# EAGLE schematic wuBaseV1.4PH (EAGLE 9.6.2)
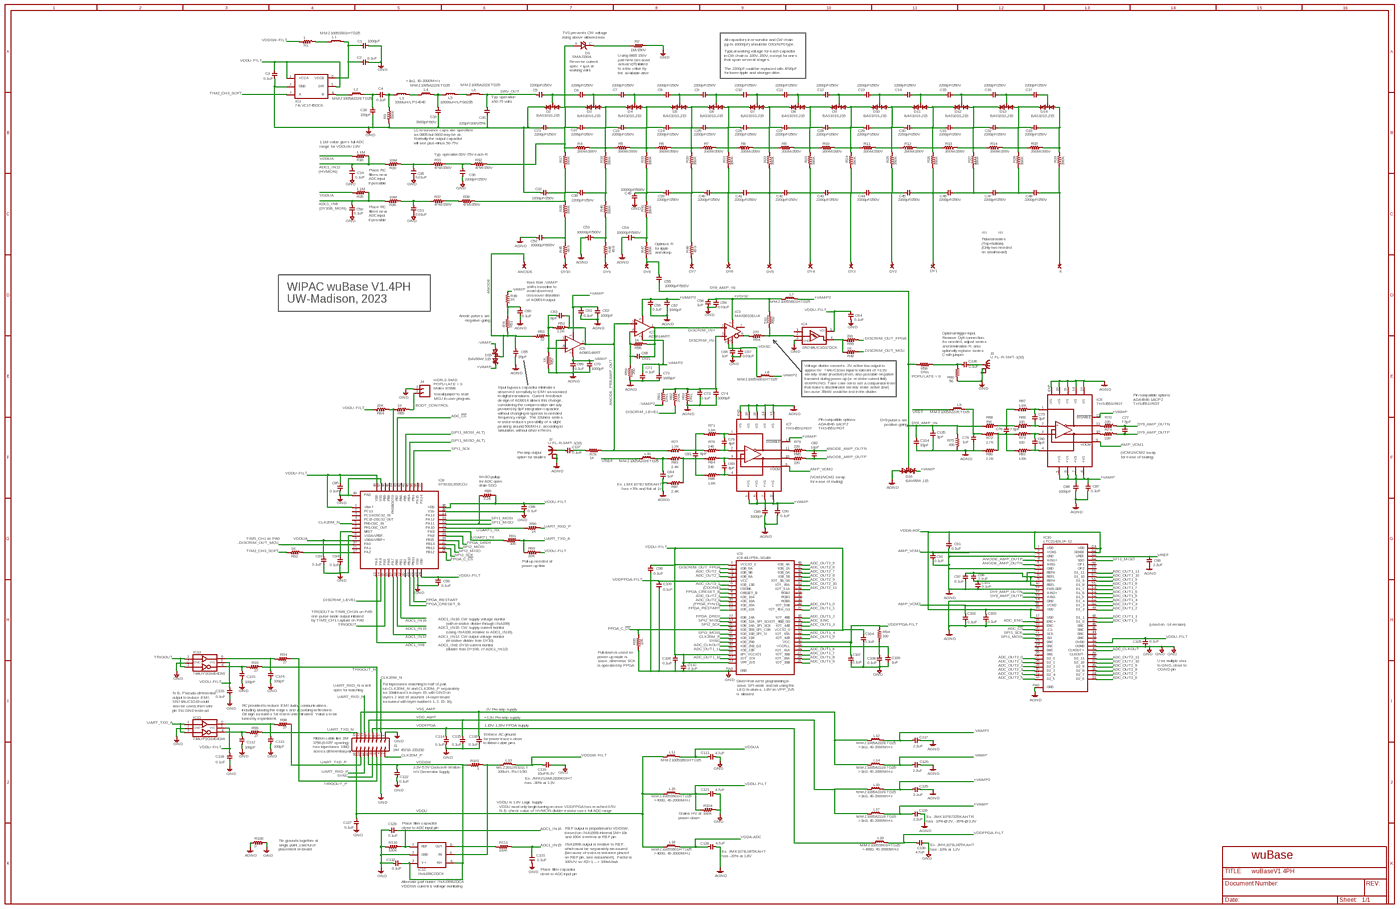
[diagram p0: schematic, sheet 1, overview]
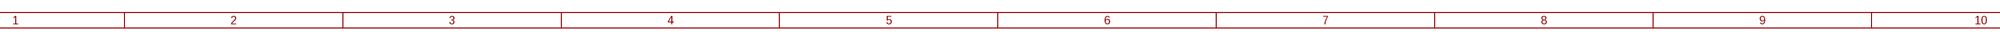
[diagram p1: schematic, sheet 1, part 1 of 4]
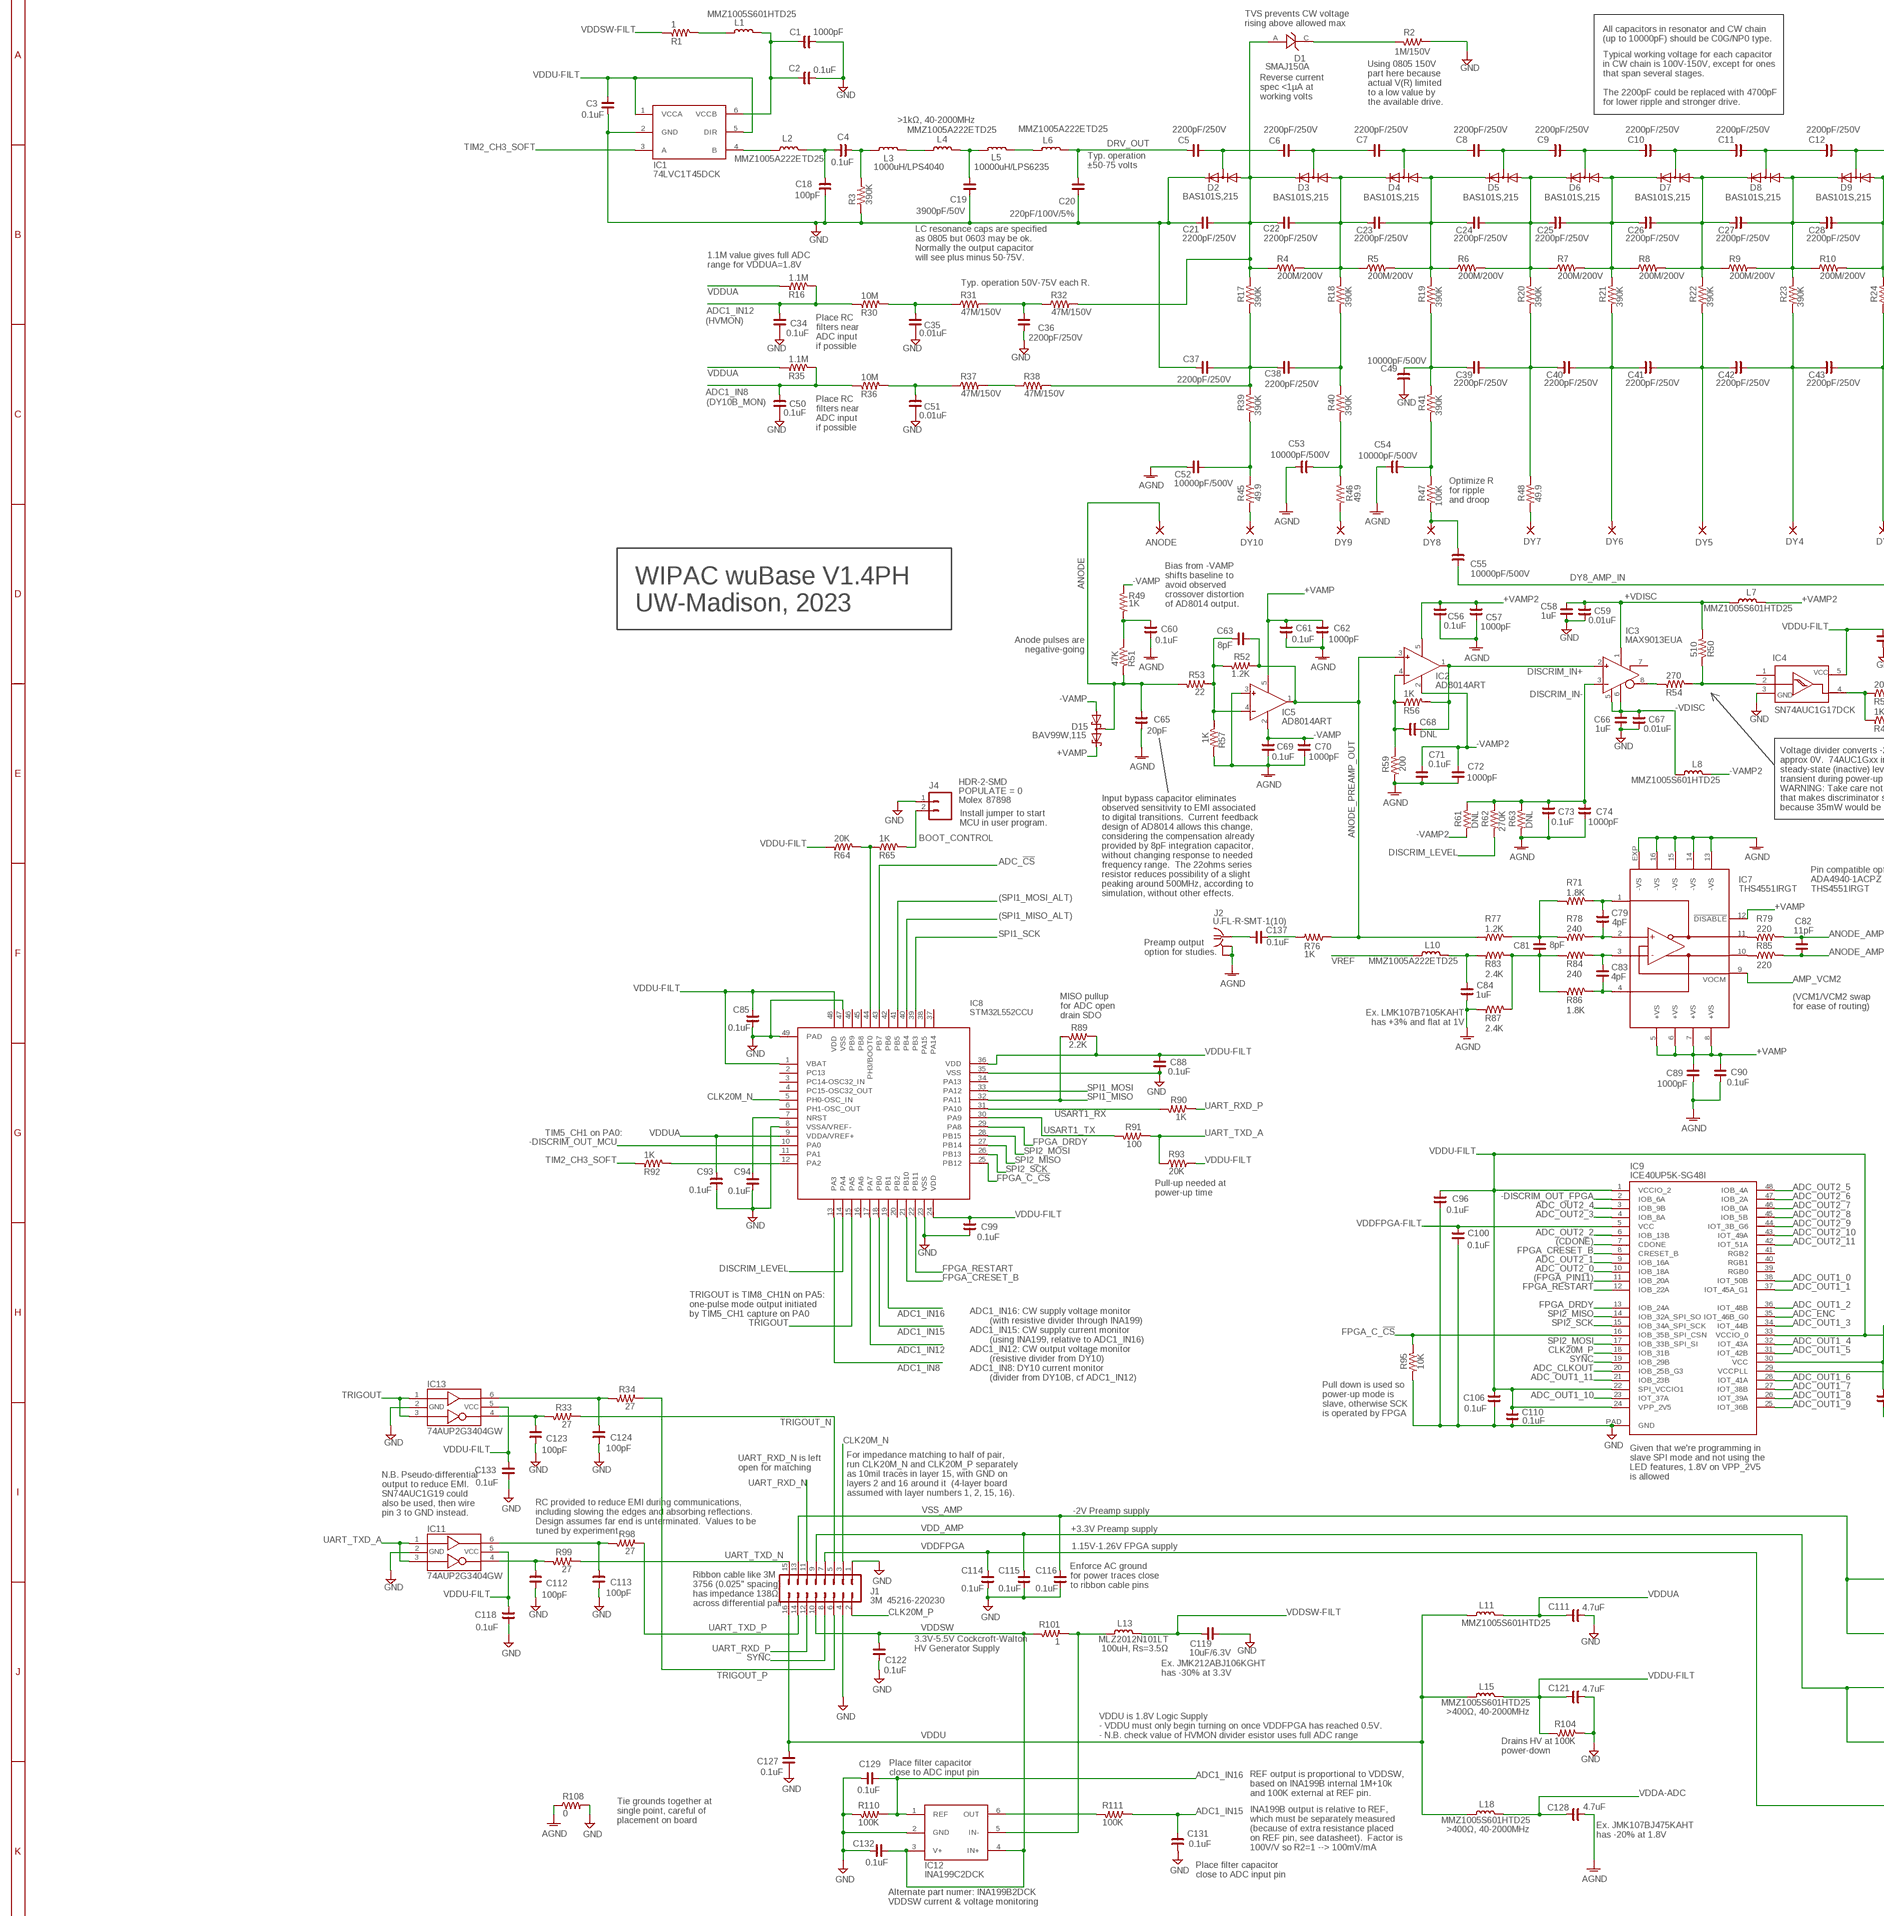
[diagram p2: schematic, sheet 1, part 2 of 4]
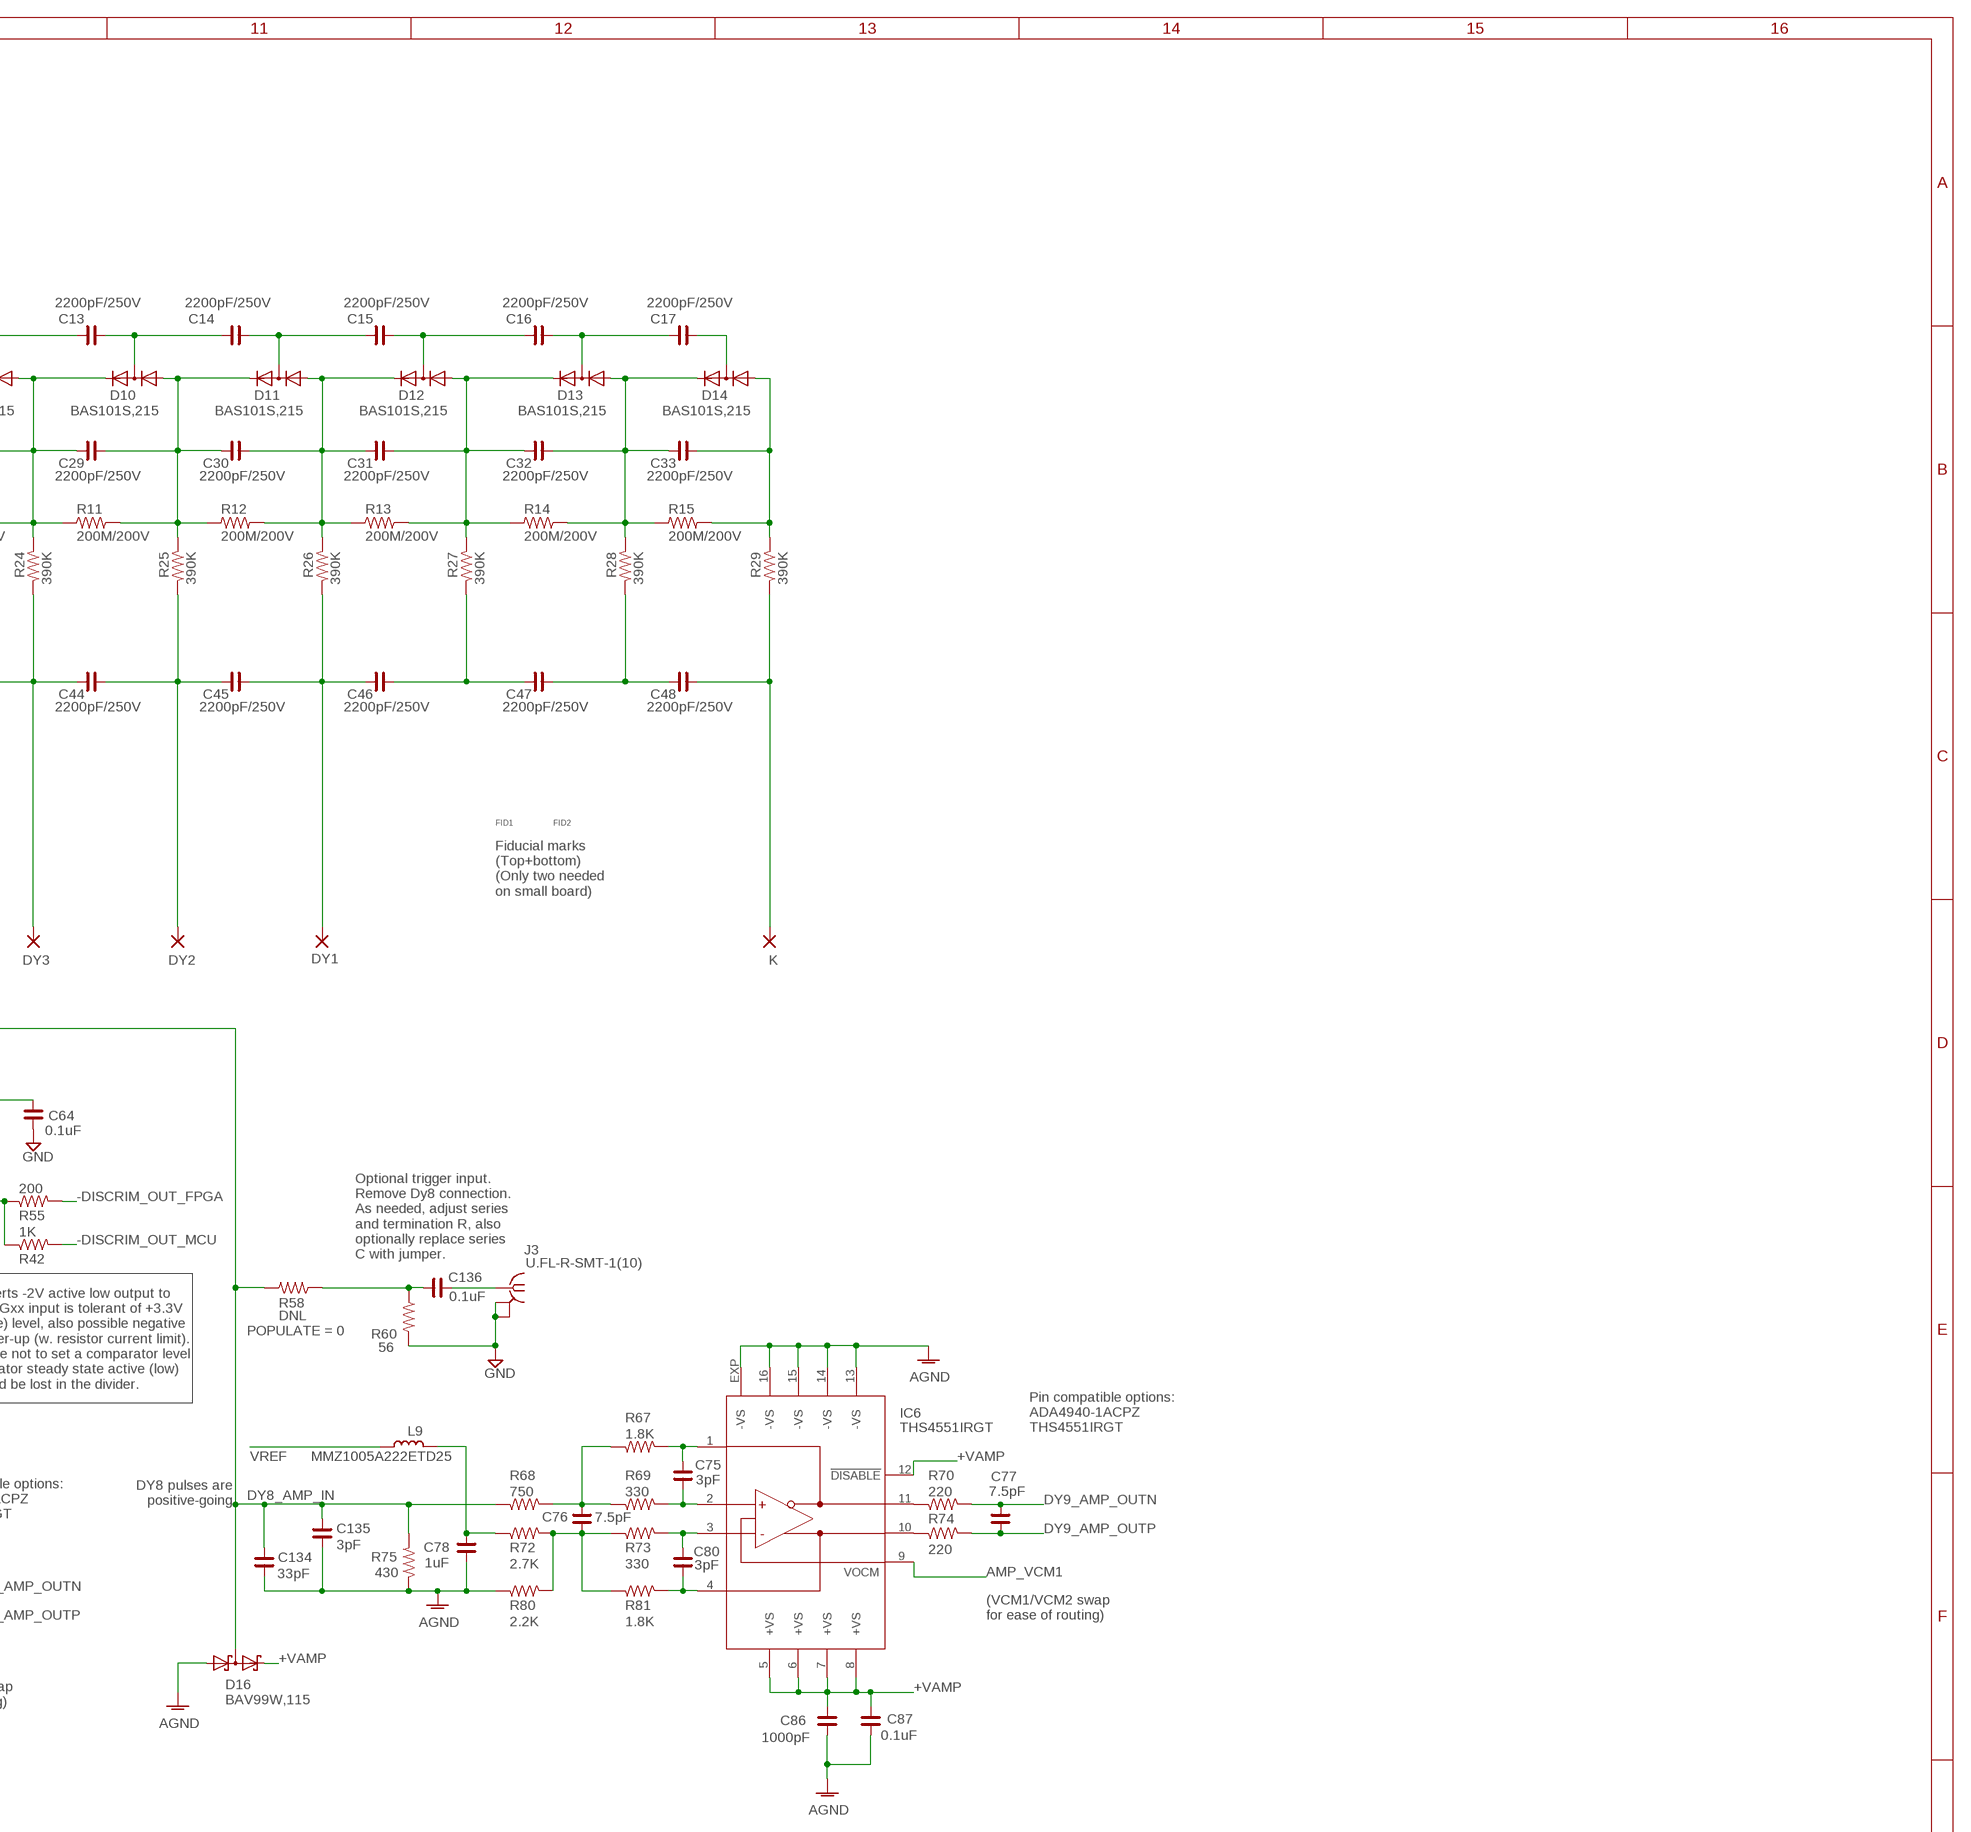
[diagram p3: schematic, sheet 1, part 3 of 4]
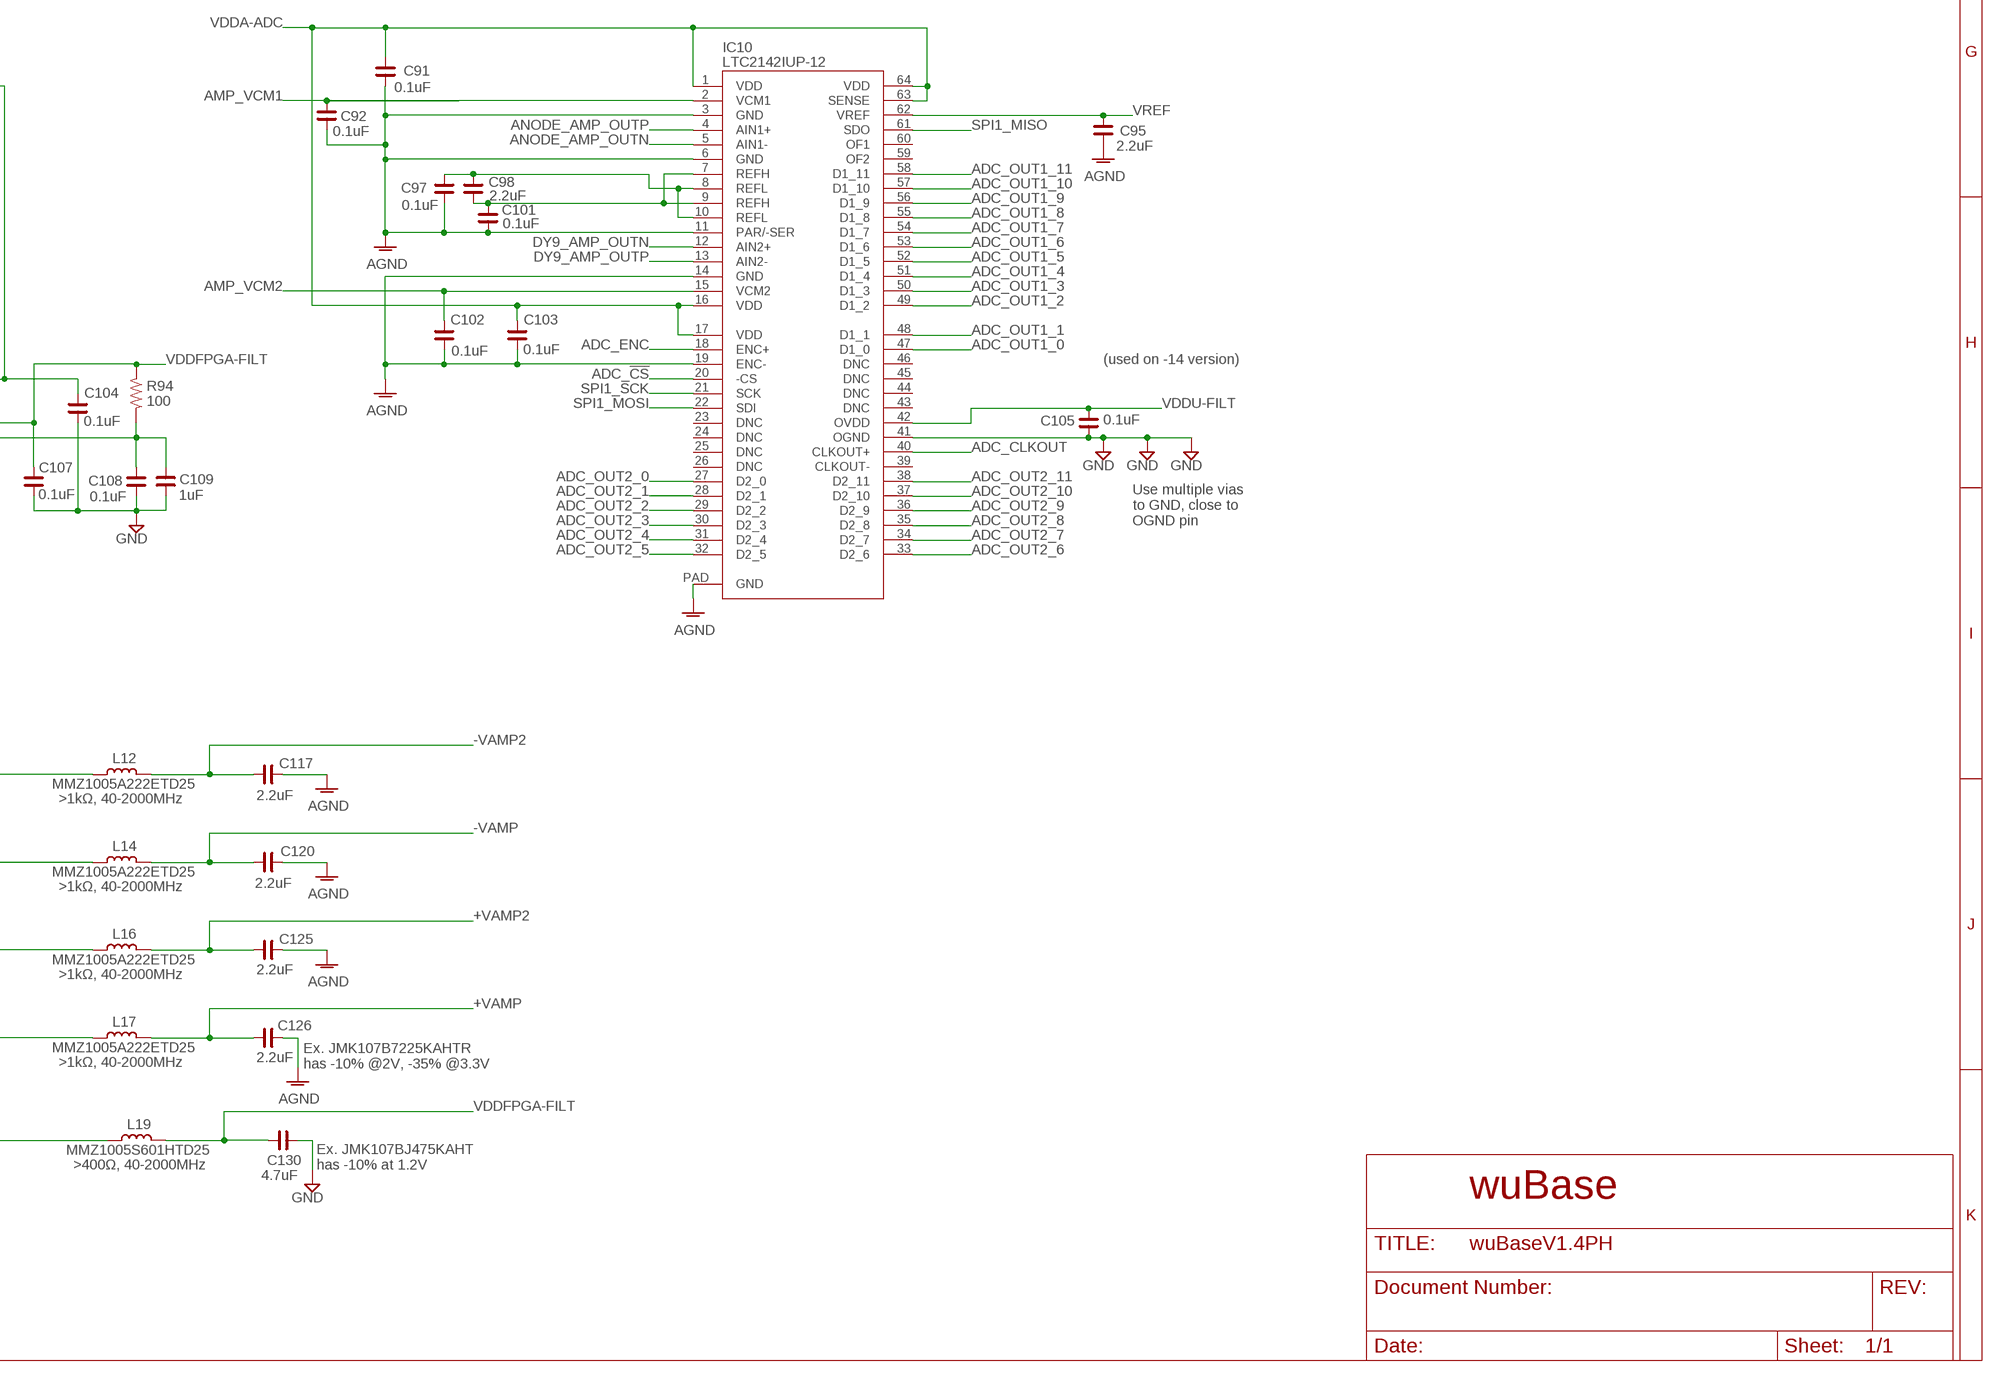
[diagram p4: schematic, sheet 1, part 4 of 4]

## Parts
ANODE  PAD-0430-BARE  [0430-BARE]
C1  1000pF  C_0402  [C0402]
C2  0.1uF  C_0402  [C0402]
C3  0.1uF  C_0402  [C0402]
C4  0.1uF  C_0402HV  [C0402-HV]
C5  2200pF/250V  C_0805HV  [C0805-HV]
C6  2200pF/250V  C_0805HV  [C0805-HV]
C7  2200pF/250V  C_0805HV  [C0805-HV]
C8  2200pF/250V  C_0805HV  [C0805-HV]
C9  2200pF/250V  C_0805HV  [C0805-HV]
C10  2200pF/250V  C_0805HV  [C0805-HV]
C11  2200pF/250V  C_0805HV  [C0805-HV]
C12  2200pF/250V  C_0805HV  [C0805-HV]
C13  2200pF/250V  C_0805HV  [C0805-HV]
C14  2200pF/250V  C_0805HV  [C0805-HV]
C15  2200pF/250V  C_0805HV  [C0805-HV]
C16  2200pF/250V  C_0805HV  [C0805-HV]
C17  2200pF/250V  C_0805HV  [C0805-HV]
C18  100pF  C_0402HV  [C0402-HV]
C19  3900pF/50V  C_0805HV  [C0805-HV]
C20  220pF/100V/5%  C_0805HV  [C0805-HV]
C21  2200pF/250V  C_0805HV  [C0805-HV]
C22  2200pF/250V  C_0805HV  [C0805-HV]
C23  2200pF/250V  C_0805HV  [C0805-HV]
C24  2200pF/250V  C_0805HV  [C0805-HV]
C25  2200pF/250V  C_0805HV  [C0805-HV]
C26  2200pF/250V  C_0805HV  [C0805-HV]
C27  2200pF/250V  C_0805HV  [C0805-HV]
C28  2200pF/250V  C_0805HV  [C0805-HV]
C29  2200pF/250V  C_0805HV  [C0805-HV]
C30  2200pF/250V  C_0805HV  [C0805-HV]
C31  2200pF/250V  C_0805HV  [C0805-HV]
C32  2200pF/250V  C_0805HV  [C0805-HV]
C33  2200pF/250V  C_0805HV  [C0805-HV]
C34  0.1uF  C_0402  [C0402]
C35  0.01uF  C_0402  [C0402]
C36  2200pF/250V  C_0805HV  [C0805-HV]
C37  2200pF/250V  C_0805HV  [C0805-HV]
C38  2200pF/250V  C_0805HV  [C0805-HV]
C39  2200pF/250V  C_0805HV  [C0805-HV]
C40  2200pF/250V  C_0805HV  [C0805-HV]
C41  2200pF/250V  C_0805HV  [C0805-HV]
C42  2200pF/250V  C_0805HV  [C0805-HV]
C43  2200pF/250V  C_0805HV  [C0805-HV]
C44  2200pF/250V  C_0805HV  [C0805-HV]
C45  2200pF/250V  C_0805HV  [C0805-HV]
C46  2200pF/250V  C_0805HV  [C0805-HV]
C47  2200pF/250V  C_0805HV  [C0805-HV]
C48  2200pF/250V  C_0805HV  [C0805-HV]
C49  10000pF/500V  C_1206HV  [C1206-HV]
C50  0.1uF  C_0402  [C0402]
C51  0.01uF  C_0402  [C0402]
C52  10000pF/500V  C_1206HV  [C1206-HV]
C53  10000pF/500V  C_1206HV  [C1206-HV]
C54  10000pF/500V  C_1206HV  [C1206-HV]
C55  10000pF/500V  C_1206HV  [C1206-HV]
C56  0.1uF  C_0402  [C0402]
C57  1000pF  C_0402  [C0402]
C58  1uF  C_0603  [C0603]
C59  0.01uF  C_0402  [C0402]
C60  0.1uF  C_0402  [C0402]
C61  0.1uF  C_0402  [C0402]
C62  1000pF  C_0402  [C0402]
C63  8pF  C_0402  [C0402]
C64  0.1uF  C_0402  [C0402]
C65  20pF  C_0402  [C0402]
C66  1uF  C_0603  [C0603]
C67  0.01uF  C_0402  [C0402]
C68  DNL  C_0402  [C0402]
C69  0.1uF  C_0402  [C0402]
C70  1000pF  C_0402  [C0402]
C71  0.1uF  C_0402  [C0402]
C72  1000pF  C_0402  [C0402]
C73  0.1uF  C_0402  [C0402]
C74  1000pF  C_0402  [C0402]
C75  3pF  C_0402  [C0402]
C76  7.5pF  C_0402  [C0402]
C77  7.5pF  C_0402  [C0402]
C78  1uF  C_0603  [C0603]
C79  4pF  C_0402  [C0402]
C80  3pF  C_0402  [C0402]
C81  8pF  C_0402  [C0402]
C82  11pF  C_0402  [C0402]
C83  4pF  C_0402  [C0402]
C84  1uF  C_0603  [C0603]
C85  0.1uF  C_0402  [C0402]
C86  1000pF  C_0402  [C0402]
C87  0.1uF  C_0402  [C0402]
C88  0.1uF  C_0402  [C0402]
C89  1000pF  C_0402  [C0402]
C90  0.1uF  C_0402  [C0402]
C91  0.1uF  C_0402  [C0402]
C92  0.1uF  C_0402  [C0402]
C93  0.1uF  C_0402  [C0402]
C94  0.1uF  C_0402  [C0402]
C95  2.2uF  C_0603  [C0603]
C96  0.1uF  C_0402  [C0402]
C97  0.1uF  C_0402  [C0402]
C98  2.2uF  C_0603  [C0603]
C99  0.1uF  C_0402  [C0402]
C100  0.1uF  C_0402  [C0402]
C101  0.1uF  C_0402  [C0402]
C102  0.1uF  C_0402  [C0402]
C103  0.1uF  C_0402  [C0402]
C104  0.1uF  C_0402  [C0402]
C105  0.1uF  C_0402  [C0402]
C106  0.1uF  C_0402  [C0402]
C107  0.1uF  C_0402  [C0402]
C108  0.1uF  C_0402  [C0402]
C109  1uF  C_0603  [C0603]
C110  0.1uF  C_0402  [C0402]
C111  4.7uF  C_0603  [C0603]
C112  100pF  C_0402  [C0402]
C113  100pF  C_0402  [C0402]
C114  0.1uF  C_0402  [C0402]
C115  0.1uF  C_0402  [C0402]
C116  0.1uF  C_0402  [C0402]
C117  2.2uF  C_0603  [C0603]
C118  0.1uF  C_0402  [C0402]
C119  10uF/6.3V  C_0805  [C0805]
C120  2.2uF  C_0603  [C0603]
C121  4.7uF  C_0603  [C0603]
C122  0.1uF  C_0402  [C0402]
C123  100pF  C_0402  [C0402]
C124  100pF  C_0402  [C0402]
C125  2.2uF  C_0603  [C0603]
C126  2.2uF  C_0603  [C0603]
C127  0.1uF  C_0402  [C0402]
C128  4.7uF  C_0603  [C0603]
C129  0.1uF  C_0402  [C0402]
C130  4.7uF  C_0603  [C0603]
C131  0.1uF  C_0402  [C0402]
C132  0.1uF  C_0402  [C0402]
C133  0.1uF  C_0402  [C0402]
C134  33pF  C_0402  [C0402]
C135  3pF  C_0402  [C0402]
C136  0.1uF  C_0402  [C0402]
C137  0.1uF  C_0402  [C0402]
D1  SMAJ150A  SMAJXXXA-HV  [DO214AC-HV]
D2  BAS101S,215  MMBD3004S-ROUNDED  [SOT23-ROUNDED]
D3  BAS101S,215  MMBD3004S-ROUNDED  [SOT23-ROUNDED]
D4  BAS101S,215  MMBD3004S-ROUNDED  [SOT23-ROUNDED]
D5  BAS101S,215  MMBD3004S-ROUNDED  [SOT23-ROUNDED]
D6  BAS101S,215  MMBD3004S-ROUNDED  [SOT23-ROUNDED]
D7  BAS101S,215  MMBD3004S-ROUNDED  [SOT23-ROUNDED]
D8  BAS101S,215  MMBD3004S-ROUNDED  [SOT23-ROUNDED]
D9  BAS101S,215  MMBD3004S-ROUNDED  [SOT23-ROUNDED]
D10  BAS101S,215  MMBD3004S-ROUNDED  [SOT23-ROUNDED]
D11  BAS101S,215  MMBD3004S-ROUNDED  [SOT23-ROUNDED]
D12  BAS101S,215  MMBD3004S-ROUNDED  [SOT23-ROUNDED]
D13  BAS101S,215  MMBD3004S-ROUNDED  [SOT23-ROUNDED]
D14  BAS101S,215  MMBD3004S-ROUNDED  [SOT23-ROUNDED]
D15  BAV99W,115  BAV99W  [SC70-3L]
D16  BAV99W,115  BAV99W  [SC70-3L]
DY1  PAD-0430-BARE  [0430-BARE]
DY2  PAD-0430-BARE  [0430-BARE]
DY3  PAD-0430-BARE  [0430-BARE]
DY4  PAD-0430-BARE  [0430-BARE]
DY5  PAD-0430-BARE  [0430-BARE]
DY6  PAD-0430-BARE  [0430-BARE]
DY7  PAD-0430-BARE  [0430-BARE]
DY8  PAD-0430-BARE  [0430-BARE]
DY9  PAD-0430-BARE  [0430-BARE]
DY10  PAD-0430-BARE  [0430-BARE]
FID1  FIDUCIAL_0.5MM  [FIDUCIAL_0.5MM]
FID2  FIDUCIAL_0.5MM  [FIDUCIAL_0.5MM]
IC1  74LVC1T45DCK  [SC70-6L-TI]
IC2  AD8014ART  [SOT23-5]
IC3  MAX9013EUA  [MSOP8]
IC4  SN74AUC1G17DCK  [SC70-5L-TI]
IC5  AD8014ART  [SOT23-5]
IC6  THS4551IRGT  ADA4940-1ACPZ  [LFCSP16]
IC7  THS4551IRGT  ADA4940-1ACPZ  [LFCSP16]
IC8  STM32L552CCU  [UFQFPN48-STMICRO]
IC9  ICE40UP5K-SG48I  [QFN48-ICE40ULTRA]
IC10  LTC2142IUP-12  LTC2141-12UP  [QFN64-LTC214X]
IC11  74AUP2G3404GW  [SC70-6L-TI]
IC12  INA199C2DCK  INA199B2DCK  [SC70-6L-TI]
IC13  74AUP2G3404GW  [SC70-6L-TI]
J1  HDR-16  HDR-2X8-3M-45216-220230  [3M-45216-220230]
J2  COAX-2GNDU.FL  [HIROSE_U.FL-R-SMT-1]
J3  COAX-2GNDU.FL  [HIROSE_U.FL-R-SMT-1]
J4  HDR-2-SMD  [HEADER-SMD-2X1-MINIMUM]
K  PAD-0430-BARE  [0430-BARE]
L1  MMZ1005S601HTD25  L_0402  [L0402]
L2  MMZ1005A222ETD25  L_0402HV  [L0402-HV]
L3  1000uH/LPS4040  L_LPS4040-REDUCED  [LPS4040-REDUCED]
L4  MMZ1005A222ETD25  L_0402HV  [L0402-HV]
L5  10000uH/LPS6235  L_LPS6235-REDUCED  [LPS6235-REDUCED]
L6  MMZ1005A222ETD25  L_0402HV  [L0402-HV]
L7  MMZ1005S601HTD25  L_0402  [L0402]
L8  MMZ1005S601HTD25  L_0402  [L0402]
L9  MMZ1005A222ETD25  L_0402  [L0402]
L10  MMZ1005A222ETD25  L_0402  [L0402]
L11  MMZ1005S601HTD25  L_0402  [L0402]
L12  MMZ1005A222ETD25  L_0402  [L0402]
L13  MLZ2012N101LT  L_0805  [L0805]
L14  MMZ1005A222ETD25  L_0402  [L0402]
L15  MMZ1005S601HTD25  L_0402  [L0402]
L16  MMZ1005A222ETD25  L_0402  [L0402]
L17  MMZ1005A222ETD25  L_0402  [L0402]
L18  MMZ1005S601HTD25  L_0402  [L0402]
L19  MMZ1005S601HTD25  L_0402  [L0402]
R1  1  R_0402  [R0402]
R2  1M/150V  R_0805HV  [R0805-HV]
R3  390K  R_0402HV  [R0402-HV]
R4  200M/200V  R_1206HV  [R1206-HV]
R5  200M/200V  R_1206HV  [R1206-HV]
R6  200M/200V  R_1206HV  [R1206-HV]
R7  200M/200V  R_1206HV  [R1206-HV]
R8  200M/200V  R_1206HV  [R1206-HV]
R9  200M/200V  R_1206HV  [R1206-HV]
R10  200M/200V  R_1206HV  [R1206-HV]
R11  200M/200V  R_1206HV  [R1206-HV]
R12  200M/200V  R_1206HV  [R1206-HV]
R13  200M/200V  R_1206HV  [R1206-HV]
R14  200M/200V  R_1206HV  [R1206-HV]
R15  200M/200V  R_1206HV  [R1206-HV]
R16  1.1M  R_0402  [R0402]
R17  390K  R_0402HV  [R0402-HV]
R18  390K  R_0402HV  [R0402-HV]
R19  390K  R_0402HV  [R0402-HV]
R20  390K  R_0402HV  [R0402-HV]
R21  390K  R_0402HV  [R0402-HV]
R22  390K  R_0402HV  [R0402-HV]
R23  390K  R_0402HV  [R0402-HV]
R24  390K  R_0402HV  [R0402-HV]
R25  390K  R_0402HV  [R0402-HV]
R26  390K  R_0402HV  [R0402-HV]
R27  390K  R_0402HV  [R0402-HV]
R28  390K  R_0402HV  [R0402-HV]
R29  390K  R_0402HV  [R0402-HV]
R30  10M  R_0402  [R0402]
R31  47M/150V  R_0805HV  [R0805-HV]
R32  47M/150V  R_0805HV  [R0805-HV]
R33  27  R_0402  [R0402]
R34  27  R_0402  [R0402]
R35  1.1M  R_0402  [R0402]
R36  10M  R_0402  [R0402]
R37  47M/150V  R_0805HV  [R0805-HV]
R38  47M/150V  R_0805HV  [R0805-HV]
R39  390K  R_0402HV  [R0402-HV]
R40  390K  R_0402HV  [R0402-HV]
R41  390K  R_0402HV  [R0402-HV]
R42  1K  R_0402  [R0402]
R45  49.9  R_0402HV  [R0402-HV]
R46  49.9  R_0402HV  [R0402-HV]
R47  100K  R_0402HV  [R0402-HV]
R48  49.9  R_0402HV  [R0402-HV]
R49  1K  R_0402  [R0402]
R50  510  R_0402  [R0402]
R51  47K  R_0402  [R0402]
R52  1.2K  R_0402  [R0402]
R53  22  R_0402  [R0402]
R54  270  R_0402  [R0402]
R55  200  R_0402  [R0402]
R56  1K  R_0402  [R0402]
R57  1K  R_0402  [R0402]
R58  DNL  R_0402  [R0402]
R59  200  R_0402  [R0402]
R60  56  R_0402  [R0402]
R61  DNL  R_0402  [R0402]
R62  270K  R_0402  [R0402]
R63  DNL  R_0402  [R0402]
R64  20K  R_0402  [R0402]
R65  1K  R_0402  [R0402]
R67  1.8K  R_0402  [R0402]
R68  750  R_0402  [R0402]
R69  330  R_0402  [R0402]
R70  220  R_0402  [R0402]
R71  1.8K  R_0402  [R0402]
R72  2.7K  R_0402  [R0402]
R73  330  R_0402  [R0402]
R74  220  R_0402  [R0402]
R75  430  R_0402  [R0402]
R76  1K  R_0402  [R0402]
R77  1.2K  R_0402  [R0402]
R78  240  R_0402  [R0402]
R79  220  R_0402  [R0402]
R80  2.2K  R_0402  [R0402]
R81  1.8K  R_0402  [R0402]
R83  2.4K  R_0402  [R0402]
R84  240  R_0402  [R0402]
R85  220  R_0402  [R0402]
R86  1.8K  R_0402  [R0402]
R87  2.4K  R_0402  [R0402]
R89  2.2K  R_0402  [R0402]
R90  1K  R_0402  [R0402]
R91  100  R_0402  [R0402]
R92  1K  R_0402  [R0402]
R93  20K  R_0402  [R0402]
R94  100  R_0402  [R0402]
R95  10K  R_0402  [R0402]
R98  27  R_0402  [R0402]
R99  27  R_0402  [R0402]
R101  1  R_0402  [R0402]
R104  100K  R_0402  [R0402]
R108  0  R_0402  [R0402]
R110  100K  R_0402  [R0402]
R111  100K  R_0402  [R0402]

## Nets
(CDONE): IC9.7(CDONE)
(FPGA_PIN11): IC9.11(IOB_20A)
(SPI1_MISO_ALT): IC8.40(PB4)
(SPI1_MOSI_ALT): IC8.41(PB5)
+VAMP: C61.1 C62.1 C86.1 C87.1 C89.1 C90.1 C126.2 D15.2(C2) D16.2(C2) IC5.5(V+) IC6.5(+VS) IC6.6(+VS) IC6.7(+VS) IC6.8(+VS) IC6.12(!DISABLE) IC7.5(+VS) IC7.6(+VS) IC7.7(+VS) IC7.8(+VS) IC7.12(!DISABLE) L17.2
+VAMP2: C56.1 C57.1 C125.2 IC2.5(V+) L7.2 L16.2
+VDISC: C58.1 C59.1 IC3.1(VCC) L7.1 R50.2
-DISCRIM_BUFOUT: IC4.4(OUT) R42.1 R55.1
-DISCRIM_OUT: IC3.8(QBAR) R54.1
-DISCRIM_OUT_DIVIDER: IC4.2(IN) R50.1 R54.2
-DISCRIM_OUT_FPGA: IC9.2(IOB_6A) R55.2
-DISCRIM_OUT_MCU: IC8.10(PA0) R42.2
-VAMP: C69.1 C70.1 C120.2 D15.1(A1) IC5.2(V-) L14.2 R49.1
-VAMP2: C71.1 C72.1 C117.2 IC2.2(V-) L8.2 L12.2 R61.2
-VDISC: C66.1 C67.1 IC3.5(LE) IC3.6(GND) L8.1
ADC1_IN8: C50.1 IC8.13(PA3) R35.2 R36.1
ADC1_IN12: C34.1 IC8.17(PA7) R16.2 R30.1
ADC1_IN15: C131.2 IC8.18(PB0) R111.1
ADC1_IN16: C129.2 IC8.19(PB1) IC12.1(REF) R110.1
ADC_!CS: IC8.43(PB7) IC10.20(-CS)
ADC_CLKOUT: IC9.20(IOB_25B_G3) IC10.40(CLKOUT+)
ADC_ENC: IC9.35(IOT_46B_G0) IC10.18(ENC+)
ADC_OUT1_0: IC9.38(IOT_50B) IC10.47(D1_0)
ADC_OUT1_1: IC9.37(IOT_45A_G1) IC10.48(D1_1)
ADC_OUT1_2: IC9.36(IOT_48B) IC10.49(D1_2)
ADC_OUT1_3: IC9.34(IOT_44B) IC10.50(D1_3)
ADC_OUT1_4: IC9.32(IOT_43A) IC10.51(D1_4)
ADC_OUT1_5: IC9.31(IOT_42B) IC10.52(D1_5)
ADC_OUT1_6: IC9.28(IOT_41A) IC10.53(D1_6)
ADC_OUT1_7: IC9.27(IOT_38B) IC10.54(D1_7)
ADC_OUT1_8: IC9.26(IOT_39A) IC10.55(D1_8)
ADC_OUT1_9: IC9.25(IOT_36B) IC10.56(D1_9)
ADC_OUT1_10: IC9.23(IOT_37A) IC10.57(D1_10)
ADC_OUT1_11: IC9.21(IOB_23B) IC10.58(D1_11)
ADC_OUT2_0: IC9.10(IOB_18A) IC10.27(D2_0)
ADC_OUT2_1: IC9.9(IOB_16A) IC10.28(D2_1)
ADC_OUT2_2: IC9.6(IOB_13B) IC10.29(D2_2)
ADC_OUT2_3: IC9.4(IOB_8A) IC10.30(D2_3)
ADC_OUT2_4: IC9.3(IOB_9B) IC10.31(D2_4)
ADC_OUT2_5: IC9.48(IOB_4A) IC10.32(D2_5)
ADC_OUT2_6: IC9.47(IOB_2A) IC10.33(D2_6)
ADC_OUT2_7: IC9.46(IOB_0A) IC10.34(D2_7)
ADC_OUT2_8: IC9.45(IOB_5B) IC10.35(D2_8)
ADC_OUT2_9: IC9.44(IOT_3B_G6) IC10.36(D2_9)
ADC_OUT2_10: IC9.43(IOT_49A) IC10.37(D2_10)
ADC_OUT2_11: IC9.42(IOT_51A) IC10.38(D2_11)
AGND: C52.1 C53.2 C54.2 C56.2 C57.2 C60.2 C61.2 C62.2 C65.2 C69.2 C70.2 C71.2 C72.2 C73.2 C74.2 C78.2 C84.2 C86.2 C87.2 C89.2 C90.2 C91.2 C92.2 C95.2 C97.2 C101.2 C102.2 C103.2 C117.1 C120.1 C125.1 C126.1 C128.1 C134.2 C135.2 D16.1(A1) IC5.3(IN+) IC6.13(-VS) IC6.14(-VS) IC6.15(-VS) IC6.16(-VS) IC6.EXP(-VS) IC7.13(-VS) IC7.14(-VS) IC7.15(-VS) IC7.16(-VS) IC7.EXP(-VS) IC10.3(GND) IC10.6(GND) IC10.11(PAR/-SER) IC10.14(GND) IC10.19(ENC-) IC10.PAD(GND) J2.2(GND) J2.3(GND) R57.2 R59.2 R63.2 R75.1 R80.1 R87.1 R108.1
AMP1_INM: C63.1 IC5.4(IN-) R52.2 R53.1 R57.1
AMP2_INM: C68.1 IC2.4(IN-) R56.1 R59.1
AMP_VCM1: C92.1 IC6.9(VOCM) IC10.2(VCM1)
AMP_VCM2: C102.1 IC7.9(VOCM) IC10.15(VCM2)
ANODE: ANODE.P$1(P) C65.1 D15.3(C1A2) R51.2 R53.2
ANODE_AMP_OUTN: C82.1 IC10.5(AIN1-) R79.2
ANODE_AMP_OUTP: C82.2 IC10.4(AIN1+) R85.2
ANODE_PREAMP_OUT: C63.2 IC2.3(IN+) IC5.1(OUT) R52.1 R76.1 R77.1
BIAS_FILT: C60.1 R49.2 R51.1
BOOT0: IC8.44(PH3/BOOT0) R64.2 R65.1
BOOT_CONTROL: J4.2 R65.2
CH1COAX: C137.1 J2.1(SIGNAL)
CH1COAX_DC: C137.2 R76.2
CH2COAX: C136.2 J3.1(SIGNAL)
CH2COAX_DC: C136.1 R58.1 R60.1
CLK20M_N: IC8.5(PH0-OSC_IN) J1.3
CLK20M_P: IC9.18(IOB_31B) J1.2
CW_1_KB: C15.2 C16.1 D12.3(C1A2)
CW_2_1: C14.2 C15.1 D11.3(C1A2)
CW_3_2: C13.2 C14.1 D10.3(C1A2)
CW_4_3: C12.2 C13.1 D9.3(C1A2)
CW_5_4: C11.2 C12.1 D8.3(C1A2)
CW_6_5: C10.2 C11.1 D7.3(C1A2)
CW_7_6: C9.2 C10.1 D6.3(C1A2)
CW_8_7: C8.2 C9.1 D5.3(C1A2)
CW_9_8: C7.2 C8.1 D4.3(C1A2)
CW_10_9: C6.2 C7.1 D3.3(C1A2)
CW_A_10: C5.2 C6.1 D2.3(C1A2)
CW_KA_K: C17.2 D14.3(C1A2)
CW_KB_KA: C16.2 C17.1 D13.3(C1A2)
DISCRIM_IN+: C68.2 IC2.1(OUT) IC3.2(IN+) R56.2
DISCRIM_IN-: C73.1 C74.1 IC3.3(IN-) R61.1 R62.1 R63.1
DISCRIM_LEVEL: IC8.14(PA4) R62.2
DRV_FILT: C4.2 C18.1 L2.2
DRV_L1INP: C4.1 L3.2 R3.2
DRV_L1OUT: L3.1 L4.1
DRV_L2INP: C19.1 L4.2 L5.2
DRV_L2OUT: L5.1 L6.2
DRV_OUT: C5.1 C20.1 L6.1
DRV_SQUARE: IC1.4(B) L2.1
DY1: C45.2 C46.1 DY1.P$1(P) R26.2
DY1A: C30.2 C31.1 D11.1(A1) D12.2(C2) R12.2 R13.1 R26.1
DY2: C44.2 C45.1 DY2.P$1(P) R25.2
DY2A: C29.2 C30.1 D10.1(A1) D11.2(C2) R11.2 R12.1 R25.1
DY3: C43.2 C44.1 DY3.P$1(P) R24.2
DY3A: C28.2 C29.1 D9.1(A1) D10.2(C2) R10.2 R11.1 R24.1
DY4: C42.2 C43.1 DY4.P$1(P) R23.2
DY4A: C27.2 C28.1 D8.1(A1) D9.2(C2) R9.2 R10.1 R23.1
DY5: C41.2 C42.1 DY5.P$1(P) R22.2
DY5A: C26.2 C27.1 D7.1(A1) D8.2(C2) R8.2 R9.1 R22.1
DY6: C40.2 C41.1 DY6.P$1(P) R21.2
DY6A: C25.2 C26.1 D6.1(A1) D7.2(C2) R7.2 R8.1 R21.1
DY7: DY7.P$1(P) R48.2
DY7A: C24.2 C25.1 D5.1(A1) D6.2(C2) R6.2 R7.1 R20.1
DY7B: C39.2 C40.1 R20.2 R48.1
DY8: C55.1 DY8.P$1(P) R47.2
DY8_AMP_IN: C55.2 C134.1 C135.1 D16.3(C1A2) R58.2 R68.1 R75.2
DY8A: C23.2 C24.1 D4.1(A1) D5.2(C2) R5.2 R6.1 R19.1
DY8B: C39.1 C49.1 R19.2 R41.1
DY8C: C54.1 R41.2 R47.1
DY9: DY9.P$1(P) R46.2
DY9_AMP_OUTN: C77.1 IC10.12(AIN2+) R70.2
DY9_AMP_OUTP: C77.2 IC10.13(AIN2-) R74.2
DY9A: C22.2 C23.1 D3.1(A1) D4.2(C2) R4.2 R5.1 R18.1
DY9B: C38.2 R18.2 R40.1
DY9C: C53.1 R40.2 R46.1
DY10: DY10.P$1(P) R45.2
DY10A: C21.2 C22.1 D1.A D2.1(A1) D3.2(C2) R4.1 R17.1 R32.2
DY10B: C37.2 C38.1 R17.2 R38.2 R39.1
DY10B_MON_A: R37.2 R38.1
DY10B_MON_B: C51.1 R36.2 R37.1
DY10C: C52.2 R39.2 R45.1
FPGA_C_!CS: IC8.25(PB12) IC9.16(IOB_35B_SPI_CSN) R95.1
FPGA_CRESET_B: IC8.21(PB10) IC9.8(CRESET_B)
FPGA_DRDY: IC8.29(PA8) IC9.13(IOB_24A)
FPGA_RESTART: IC8.22(PB11) IC9.12(IOB_22A)
GND: C1.1 C2.1 C3.1 C18.2 C19.2 C20.2 C21.1 C34.2 C35.2 C36.2 C37.1 C49.2 C50.2 C51.2 C58.2 C59.2 C64.1 C66.2 C67.2 C85.2 C88.2 C93.2 C94.2 C96.2 C99.2 C100.2 C104.2 C105.2 C106.2 C107.2 C108.2 C109.2 C110.2 C111.1 C112.2 C113.2 C114.2 C115.2 C116.2 C118.2 C119.2 C121.1 C122.2 C123.2 C124.2 C127.2 C129.1 C130.2 C131.1 C132.1 C133.2 D2.2(C2) IC1.2(GND) IC4.3(GND) IC8.8(VSSA/VREF-) IC8.23(VSS) IC8.35(VSS) IC8.47(VSS) IC8.49(PAD) IC9.PAD(GND) IC10.41(OGND) IC11.2(GND) IC12.2(GND) IC13.2(GND) J1.1 J1.4 J3.2(GND) J3.3(GND) J4.1 R2.1 R3.1 R60.2 R95.2 R104.1 R108.2 R110.2
HVMON_A: C36.1 R31.2 R32.1
HVMON_B: C35.1 R30.2 R31.1
K: C48.2 K.P$1(P) R29.2
K-DY1-AA: C32.2 C33.1 D13.1(A1) D14.2(C2) R14.2 R15.1 R28.1
K-DY1-AB: C47.2 C48.1 R28.2
K-DY1-BA: C31.2 C32.1 D12.1(A1) D13.2(C2) R13.2 R14.1 R27.1
K-DY1-BB: C46.2 C47.1 R27.2
KA: C33.2 D14.1(A1) R15.2 R29.1
N$11: C79.2 IC7.2(+IN) R78.2
N$15: C83.1 IC7.3(-IN) R84.2
N$16: C81.2 R83.2 R84.1 R86.1 R87.2
N$17: C81.1 R71.1 R77.2 R78.1
N$18: C79.1 IC7.1(-FB) R71.2
N$19: C83.2 IC7.4(+FB) R86.2
N$22: IC7.11(-OUT) R79.1
N$23: IC7.10(+OUT) R85.1
N$25: C75.2 IC6.2(+IN) R69.2
N$26: C80.1 IC6.3(-IN) R73.2
N$27: C76.1 R67.1 R68.2 R69.1
N$28: C76.2 R72.2 R73.1 R80.2 R81.1
N$29: C75.1 IC6.1(-FB) R67.2
N$30: C80.2 IC6.4(+FB) R81.2
N$33: IC6.11(-OUT) R70.1
N$34: IC6.10(+OUT) R74.1
NRST: C94.1 IC8.7(NRST)
REFH: C98.2 C101.1 IC10.7(REFH) IC10.9(REFH)
REFL: C97.1 C98.1 IC10.8(REFL) IC10.10(REFL)
SPI1_MISO: IC8.32(PA11) IC10.61(SDO) R89.2
SPI1_MOSI: IC8.33(PA12) IC10.22(SDI)
SPI1_SCK: IC8.39(PB3) IC10.21(SCK)
SPI2_MISO: IC8.27(PB14) IC9.14(IOB_32A_SPI_SO)
SPI2_MOSI: IC8.28(PB15) IC9.17(IOB_33B_SPI_SI)
SPI2_SCK: IC8.26(PB13) IC9.15(IOB_34A_SPI_SCK)
SYNC: IC9.19(IOB_29B) J1.8
TIM2_CH3: IC8.12(PA2) R92.2
TIM2_CH3_SOFT: IC1.3(A) R92.1
TRIGOUT: IC8.15(PA5) IC13.1(1A) IC13.3(2A)
TRIGOUT_N: J1.5 R33.1
TRIGOUT_NA: C123.1 IC13.4(2Y) R33.2
TRIGOUT_P: J1.6 R34.1
TRIGOUT_PA: C124.1 IC13.6(1Y) R34.2
TVS_OUT: D1.C R2.2
UART_RXD_N: J1.11
UART_RXD_P: J1.12 R90.1
UART_TXD_A: IC11.1(1A) IC11.3(2A) R91.1 R93.1
UART_TXD_N: J1.15 R99.1
UART_TXD_NA: C112.1 IC11.4(2Y) R99.2
UART_TXD_P: J1.14 R98.1
UART_TXD_PA: C113.1 IC11.6(1Y) R98.2
USART1_RX: IC8.31(PA10) R90.2
USART1_TX: IC8.30(PA9) R91.2
VCCPLL: C108.1 C109.1 IC9.29(VCCPLL) R94.2
VDD_AMP: C115.1 J1.9 L16.1 L17.1
VDDA-ADC: C91.1 C103.1 C128.2 IC10.1(VDD) IC10.16(VDD) IC10.17(VDD) IC10.63(SENSE) IC10.64(VDD) L18.2
VDDFPGA: C114.1 J1.7 L19.1
VDDFPGA-FILT: C100.1 C107.1 C130.1 IC9.5(VCC) IC9.30(VCC) L19.2 R94.1
VDDSW: C122.1 C132.2 IC12.3(V+) IC12.4(IN+) J1.10 R101.2
VDDSW-FILT: C119.1 L13.2 R1.1
VDDSW-FILT-RL: L1.2 R1.2
VDDSW-FINAL: C1.2 C2.2 IC1.6(VCCB) L1.1
VDDSW-RL: IC12.5(IN-) L13.1 R101.1
VDDSW_IMON: IC12.6(OUT) R111.2
VDDU: C127.1 J1.16 L11.1 L15.1 L18.1
VDDU-FILT: C3.2 C64.2 C85.1 C88.1 C96.1 C99.1 C104.1 C105.1 C106.1 C110.1 C118.1 C121.2 C133.1 IC1.1(VCCA) IC1.5(DIR) IC4.5(VCC) IC8.1(VBAT) IC8.24(VDD) IC8.36(VDD) IC8.48(VDD) IC9.1(VCCIO_2) IC9.22(SPI_VCCIO1) IC9.24(VPP_2V5) IC9.33(VCCIO_0) IC10.42(OVDD) IC11.5(VCC) IC13.5(VCC) L15.2 R64.1 R89.1 R93.2 R104.2
VDDUA: C93.1 C111.2 IC8.9(VDDA/VREF+) L11.2 R16.1 R35.1
VREF: C95.1 IC10.62(VREF) L9.1 L10.1
VREF_FILT1: C84.1 L10.2 R83.1
VREF_FILT2: C78.1 L9.2 R72.1
VSS_AMP: C116.1 J1.13 L12.1 L14.1
Unconnected: IC3.7(Q) IC4.1(NC) IC8.2(PC13) IC8.3(PC14-OSC32_IN) IC8.4(PC15-OSC32_OUT) IC8.6(PH1-OSC_OUT) IC8.11(PA1) IC8.16(PA6) IC8.20(PB2) IC8.34(PA13) IC8.37(PA14) IC8.38(PA15) IC8.42(PB6) IC8.45(PB8) IC8.46(PB9) IC9.39(RGB0) IC9.40(RGB1) IC9.41(RGB2) IC10.23(DNC) IC10.24(DNC) IC10.25(DNC) IC10.26(DNC) IC10.39(CLKOUT-) IC10.43(DNC) IC10.44(DNC) IC10.45(DNC) IC10.46(DNC) IC10.59(OF2) IC10.60(OF1)

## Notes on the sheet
- TVS prevents CW voltage
  rising above allowed max
- All capacitors in resonator and CW chain
  (up to 10000pF) should be C0G/NP0 type.
- Reverse current 
  spec <1µA at 
  working volts
- Using 0805 150V
  part here because
  actual V(R) limited
  to a low value by
  the available drive.
- Typical working voltage for each capacitor
  in CW chain is 100V-150V, except for ones
  that span several stages.
  
  The 2200pF could be replaced with 4700pF
  for lower ripple and stronger drive.
- >1kΩ, 40-2000MHz
- Typ. operation
  ±50-75 volts
- LC resonance caps are specified 
  as 0805 but 0603 may be ok.
  Normally the output capacitor 
  will see plus minus 50-75V.
- 1.1M value gives full ADC 
  range for VDDUA=1.8V
- Typ. operation 50V-75V each R.
- (HVMON)
- Place RC
  filters near
  ADC input
  if possible
- (DY10B_MON)
- Place RC
  filters near
  ADC input
  if possible
- Fiducial marks
  (Top+bottom)
  (Only two needed
  on small board)
- Optimize R
  for ripple
  and droop
- Bias from -VAMP
  shifts baseline to
  avoid observed
  crossover distortion 
  of AD8014 output.
- WIPAC wuBase V1.4PH
  UW-Madison, 2023
- Anode pulses are
  negative-going
- Optional trigger input.  
  Remove Dy8 connection.
  As needed, adjust series
  and termination R, also
  optionally replace series
  C with jumper.
- Voltage divider converts -2V active low output to 
  approx 0V.  74AUC1Gxx input is tolerant of +3.3V 
  steady-state (inactive) level, also possible negative 
  transient during power-up (w. resistor current limit).
  WARNING: Take care not to set a comparator level 
  that makes discriminator steady state active (low) 
  because 35mW would be lost in the divider.
- Install jumper to start 
  MCU in user program.
- Pin compatible options:
  ADA4940-1ACPZ
  THS4551IRGT
- DY8 pulses are
  positive-going
- Pin compatible options:
  ADA4940-1ACPZ
  THS4551IRGT
- Input bypass capacitor eliminates
  observed sensitivity to EMI associated
  to digital transitions.  Current feedback
  design of AD8014 allows this change,
  considering the compensation already
  provided by 8pF integration capacitor,
  without changing response to needed
  frequency range.  The 22ohms series
  resistor reduces possibility of a slight
  peaking around 500MHz, according to
  simulation, without other effects.
- Preamp output
  option for studies.
- (VCM1/VCM2 swap
  for ease of routing)
- Ex. LMK107B7105KAHT
  has +3% and flat at 1V
- (VCM1/VCM2 swap
  for ease of routing)
- MISO pullup
  for ADC open
  drain SDO
- TIM5_CH1 on PA0:
- Pull-up needed at
  power-up time
- ADC1_IN16: CW supply voltage monitor
          (with resistive divider through INA199)
  ADC1_IN15: CW supply current monitor 
          (using INA199, relative to ADC1_IN16)
  ADC1_IN12: CW output voltage monitor
          (resistive divider from DY10)
  ADC1_IN8: DY10 current monitor
          (divider from DY10B, cf ADC1_IN12)
- TRIGOUT is TIM8_CH1N on PA5:
  one-pulse mode output initiated
  by TIM5_CH1 capture on PA0
- (used on -14 version)
- Pull down is used so
  power-up mode is 
  slave, otherwise SCK
  is operated by FPGA
- Use multiple vias
  to GND, close to
  OGND pin
- UART_RXD_N is left
  open for matching
- Given that we're programming in
  slave SPI mode and not using the
  LED features, 1.8V on VPP_2V5
  is allowed
- For impedance matching to half of pair,
  run CLK20M_N and CLK20M_P separately
  as 10mil traces in layer 15, with GND on
  layers 2 and 16 around it  (4-layer board
  assumed with layer numbers 1, 2, 15, 16).
- -2V Preamp supply
- N.B. Pseudo-differential
  output to reduce EMI.
  SN74AUC1G19 could
  also be used, then wire
  pin 3 to GND instead.
- +3.3V Preamp supply
- RC provided to reduce EMI during communications,
  including slowing the edges and absorbing reflections.
  Design assumes far end is unterminated.  Values to be
  tuned by experiment.
- 1.15V-1.26V FPGA supply
- Enforce AC ground
  for power traces close
  to ribbon cable pins
- >1kΩ, 40-2000MHz
- Ribbon cable like 3M
  3756 (0.025" spacing)
  has impedance 138Ω 
  across differential pair
- 3.3V-5.5V Cockcroft-Walton
  HV Generator Supply
- 100uH, Rs=3.5Ω | >1kΩ, 40-2000MHz
- Ex. JMK212ABJ106KGHT
  has -30% at 3.3V
- >1kΩ, 40-2000MHz
- VDDU is 1.8V Logic Supply
  - VDDU must only begin turning on once VDDFPGA has reached 0.5V.
  - N.B. check value of HVMON divider esistor uses full ADC range
- >400Ω, 40-2000MHz
- Drains HV at
  power-down
- >1kΩ, 40-2000MHz
- Ex. JMK107B7225KAHTR
  has -10% @2V, -35% @3.3V
- Place filter capacitor
  close to ADC input pin
- REF output is proportional to VDDSW, 
  based on INA199B internal 1M+10k
  and 100K external at REF pin.
- Tie grounds together at 
  single point, careful of 
  placement on board
- >400Ω, 40-2000MHz
- Ex. JMK107BJ475KAHT
  has -10% at 1.2V
- >400Ω, 40-2000MHz
- Ex. JMK107BJ475KAHT
  has -20% at 1.8V
- wuBase
- INA199B output is relative to REF, 
  which must be separately measured 
  (because of extra resistance placed 
  on REF pin, see datasheet).  Factor is
  100V/V so R2=1 --> 100mV/mA
- Place filter capacitor
  close to ADC input pin
- Alternate part numer: INA199B2DCK
  VDDSW current & voltage monitoring

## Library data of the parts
ANODE DY1-DY10 K = chw:PAD: Wire or pin pad
C1 C57 C62 C70 C72 C74 C86 C89 = chw:C_: Capacitor; MPN: GCM155R71H102KA37D; POPULATE: 1
C2-C4 C34 C50 C56 C60 C61 C64 C69 C71 C73 C85 C87 C88 C90-C94 C96 C97 C99-C108 C110 C114-C116 C118 C122 C127 C129 C131-C133 C136 C137 = chw:C_: Capacitor; MPN: GCM155R71C104KA55D; POPULATE: 1
C5-C17 C21-C33 C36-C48 = chw:C_: Capacitor; MPN: C0805C222JAGACAUTO; POPULATE: 1
C18 C112 C113 C123 C124 = chw:C_: Capacitor; MPN: C0402C101J3GACAUTO; POPULATE: 1
C19 = chw:C_: Capacitor; MPN: CGA4C2C0G1H392J060AA; POPULATE: 1
C20 = chw:C_: Capacitor; MPN: C0805C221J1GACAUTO; POPULATE: 1
C35 C51 C59 C67 = chw:C_: Capacitor; MPN: CGA2B2X5R1E103K050BA; POPULATE: 1
C49 C52-C55 = chw:C_: Capacitor; MPN: CGA5L4NP02J103J160AA; POPULATE: 1
C58 C66 C78 C84 C109 = chw:C_: Capacitor; MPN: LMK107B7105KAHT; POPULATE: 1
C63 C81 = chw:C_: Capacitor; MPN: GCM1555C1H8R0BA16D; POPULATE: 1
C65 = chw:C_: Capacitor; MPN: GCM1555C1H200JA16D; POPULATE: 1
C68 = chw:C_: Capacitor; POPULATE: 0
C75 C80 C135 = chw:C_: Capacitor; MPN: GCM1555C1H3R0BA16D; POPULATE: 1
C76 C77 = chw:C_: Capacitor; MPN: GCQ1555C1H7R5BB01D; POPULATE: 1
C79 C83 = chw:C_: Capacitor; MPN: GCM1555C1H4R0BA16D; POPULATE: 1
C82 = chw:C_: Capacitor; MPN: GCM1555C1H110FA16D; POPULATE: 1
C95 C98 C117 C120 C125 C126 = chw:C_: Capacitor; MPN: CGA3E1X7R0J225K080AC; POPULATE: 1
C111 C121 C128 C130 = chw:C_: Capacitor; MPN: JMK107BJ475KAHT; POPULATE: 1
C119 = chw:C_: Capacitor; MPN: C0805C106K8PACTU; POPULATE: 1
C134 = chw:C_: Capacitor; MPN: GCM1555C1H330FA16D; POPULATE: 1
D1 = chw:SMAJ*A: TVS Diode, unidirectional; MPN: SMAJ150A
D2-D14 = chw:MMBD3004S; MPN: BAS101S,215; POPULATE: 1
D15 D16 = chw:BAV99: Dual Schottky Diodes; MPN: BAV99W,115; POPULATE: 1
FID1 FID2 = chw:FIDUCIAL: Library: MF_Aesthetics; HOUSEPART: NO; POPULATE: 0
IC1 = chw:74*1T45: 74*1T45 Level Translator; MPN: 74LVC1T45GW-Q100H; POPULATE: 1
IC2 IC5 = chw:AD8014: AD8014 Op amp, 400MHz, 1.15mA, 3.5nV/sqrtHz; MPN: AD8014ARTZ-REEL7; POPULATE: 1
IC3 = chw:MAX9013: Comparator with differential output and latch enable; MPN: MAX9013EUA+; POPULATE: 1
IC4 = chw:SN74*1G17: Schmitt trigger buffer; MPN: SN74AUC1G17DCKR
IC6 IC7 = chw:ADA4940-1: Ultralow Power, Low Distortion Fully Differential ADC Driver; MPN: THS4551IRGTR; POPULATE: 1
IC8 = chw:STM32L552C: STM32L552 ARM Cortex-M33 MCU+FPU; MPN: STM32L552CCU6; POPULATE: 1
IC9 = chw:ICE40UP5K-SG48I: iCE40 Ultra FPGA SG48 version; MPN: ICE40UP5K-SG48I; POPULATE: 1
IC10 = chw:LTC2141-12; MPN: LTC2141IUP-12; POPULATE: 1
IC11 IC13 = chw:74*2G3404: Buffer plus inverter; MPN: 74AUP2G3404GW,125; POPULATE: 1
IC12 = chw:INA199: INA199 Low or High-Side Current Shunt Monitor; MPN: INA199C2DCKR; POPULATE: 1
J1 = chw:HDR-2X8; MFG: 3M; MPN: 45216-220230; POPULATE: 1
J2 J3 = chw:COAX-2GND; MPN: U.FL-R-SMT-1(10); POPULATE: 1
J4 = chw:HDR-2: Header or Screw Terminal Block; MFG: Molex; MPN: 87898; POPULATE: 0
L1 L7 L8 L11 L15 L18 L19 = chw:L_; MPN: MMZ1005S601ETD25; POPULATE: 1
L2 L4 L6 L9 L10 L12 L14 L16 L17 = chw:L_; MPN: MMZ1005A222ETD25; POPULATE: 1
L3 = chw:L_; MPN: LPS4040-105MRC; POPULATE: 1
L5 = chw:L_; MPN: LPS6235-106MRC; POPULATE: 1
L13 = chw:L_; MPN: MLZ2012N101LTD25; POPULATE: 1
R1 R101 = chw:R_: Resistor; MPN: AC0402FR-071RL; POPULATE: 1
R2 = chw:R_: Resistor; MPN: AC0805FR-071ML; POPULATE: 1
R3 R17-R29 R39-R41 = chw:R_: Resistor; MPN: AC0402FR-07390KL; POPULATE: 1
R4-R15 = chw:R_: Resistor; MPN: CRCW1206200MJPEAHR; POPULATE: 1
R16 R35 = chw:R_: Resistor; MPN: AC0402FR-071M1L; POPULATE: 1
R30 R36 = chw:R_: Resistor; MPN: AC0402FR-0710ML; POPULATE: 1
R31 R32 R37 R38 = chw:R_: Resistor; MPN: RC0805JR-0747ML; POPULATE: 1
R33 R34 R98 R99 = chw:R_: Resistor; MPN: AC0402FR-0727RL; POPULATE: 1
R42 R49 R56 R57 R65 R76 R90 R92 = chw:R_: Resistor; MPN: AC0402FR-071KL; POPULATE: 1
R45 R46 R48 = chw:R_: Resistor; MPN: AC0402FR-0749R9L; POPULATE: 1
R47 R104 R110 R111 = chw:R_: Resistor; MPN: AC0402FR-07100KL; POPULATE: 1
R50 = chw:R_: Resistor; MPN: AC0402FR-07510RL; POPULATE: 1
R51 = chw:R_: Resistor; MPN: AC0402FR-0747KL; POPULATE: 1
R52 R77 = chw:R_: Resistor; MPN: AC0402FR-071K2L; POPULATE: 1
R53 = chw:R_: Resistor; MPN: AC0402FR-0722RL; POPULATE: 1
R54 = chw:R_: Resistor; MPN: AC0402FR-07270RL; POPULATE: 1
R55 R59 = chw:R_: Resistor; MPN: AC0402FR-07200RL; POPULATE: 1
R58 R61 R63 = chw:R_: Resistor; POPULATE: 0
R60 = chw:R_: Resistor; MPN: AC0402FR-0756RL; POPULATE: 1
R62 = chw:R_: Resistor; MPN: AC0402FR-07270KL; POPULATE: 1
R64 R93 = chw:R_: Resistor; MPN: AC0402FR-0720KL; POPULATE: 1
R67 R71 R81 R86 = chw:R_: Resistor; MPN: AC0402FR-071K8L; POPULATE: 1
R68 = chw:R_: Resistor; MPN: AC0402FR-07750RL; POPULATE: 1
R69 R73 = chw:R_: Resistor; MPN: AC0402FR-07330RL; POPULATE: 1
R70 R74 R79 R85 = chw:R_: Resistor; MPN: AC0402FR-07220RL; POPULATE: 1
R72 = chw:R_: Resistor; MPN: AC0402FR-072K7L; POPULATE: 1
R75 = chw:R_: Resistor; MPN: AC0402FR-07430RL; POPULATE: 1
R78 R84 = chw:R_: Resistor; MPN: AC0402FR-07240RL; POPULATE: 1
R80 R89 = chw:R_: Resistor; MPN: AC0402FR-072K2L; POPULATE: 1
R83 R87 = chw:R_: Resistor; MPN: AC0402FR-072K4L; POPULATE: 1
R91 R94 = chw:R_: Resistor; MPN: AC0402FR-07100RL; POPULATE: 1
R95 = chw:R_: Resistor; MPN: AC0402FR-0710KL; POPULATE: 1
R108 = chw:R_: Resistor; MPN: RC0402JR-070RL; POPULATE: 1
